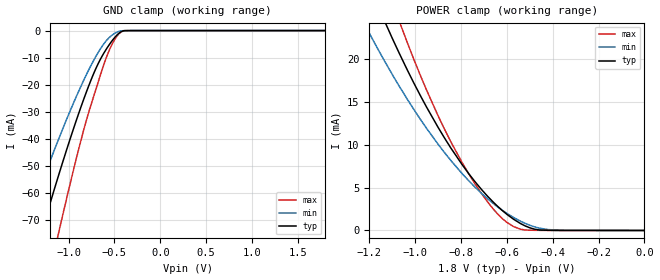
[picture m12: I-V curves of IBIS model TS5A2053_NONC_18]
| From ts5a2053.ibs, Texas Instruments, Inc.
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[Model]   TS5A2053_NONC_18
Model_type  Terminator
| variable   typ   min   max
C_comp   7.34pF   6.50pF   8.03pF
| C_tri-state   7.34pF   6.50pF   8.03pF
[Temperature Range]   40   100   -40
| Ambient temperature   25   85   -40
[Voltage range]   1.8   1.65   1.95
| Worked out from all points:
|   GND clamp passes 1 mA (typ) near -0.45 V on its own axis
|   POWER clamp passes 1 mA (typ) near -0.55 V on its own axis
[GND Clamp]
| TS5A2053_NONC_18
|   Voltage   I(typ)   I(min)   I(max)
-5.5V     -656.6mA   -514.9mA   -884.2mA
-1.495V   -98.46mA   -75.33mA   -135.4mA
-1.445V   -92.4mA    -70.58mA   -127.3mA
-1.295V   -74.61mA   -56.63mA   -103.3mA
-1.11V    -53.63mA   -40.24mA   -75.03mA
-875mV    -29.19mA   -21.3mA    -41.86mA
-750mV    -17.82mA   -12.52mA   -26.87mA
-655mV    -10.72mA   -6.852mA   -16.63mA
-570mV    -5.893mA   -3.03mA    -8.372mA
-505mV    -2.88mA    -1.184mA   -3.733mA
-435mV    -614.2uA   -158uA     -700.3uA
1.8V      377.2pA    93.4nA     3.511nA
[POWER Clamp]
| TS5A2053_NONC_18
|   Voltage   I(typ)   I(min)   I(max)
-5.5V     596.6mA    479.1mA    771.4mA
-1.23V    30.5mA     24.51mA    37.12mA
-1.2V     28.54mA    22.98mA    34.58mA
-1.135V   24.48mA    19.81mA    29.33mA
-1.07V    20.68mA    16.84mA    24.43mA
-1.035V   18.74mA    15.32mA    21.94mA
-950mV    14.36mA    11.89mA    16.34mA
-795mV    7.666mA    6.622mA    7.897mA
-685mV    4.013mA    3.717mA    3.363mA
-600mV    1.886mA    1.993mA    946.5uA
-460mV    62.87uA    280.1uA    16.8uA
-95.1fV   377.2pA    2.603nA    8.711nA
